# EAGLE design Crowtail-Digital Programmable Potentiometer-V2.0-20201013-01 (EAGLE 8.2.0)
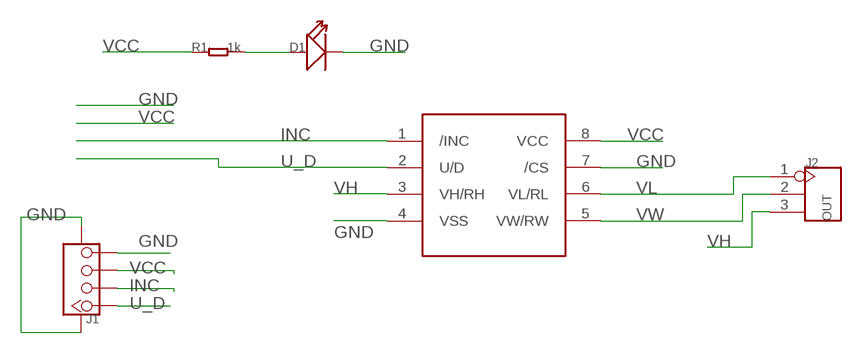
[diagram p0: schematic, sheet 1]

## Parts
D1  LED'0603'  [LED-0603]
J1  TWIG-4P-2.0-SMD-FEMALE-REINFORCE'DD'  [4P-SMD-2.0]
J2  OUT  HEADER-3P-2.54  [3P-2.54]
R1  1k  R-0603  [0603]
U1  X9C103S  [SOP8]

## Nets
GND: D1.- J1.4 J1.SS1 J1.SS2 U1.4(VSS) U1.7(/CS)
INC: J1.2 U1.1(/INC)
N$5: D1.+ R1.2
U_D: J1.1 U1.2(U/D)
VCC: J1.3 R1.1 U1.8(VCC)
VH: J2.3 U1.3(VH/RH)
VL: J2.1 U1.6(VL/RL)
VW: J2.2 U1.5(VW/RW)

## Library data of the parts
D1 = Discrete:LED*
J1 = Connector:TWIG-4P-2.0-SMD-FEMALE-REINFORCE
J2 = Connector:HEADER-3P
R1 = Discrete:R*
U1 = IC:X9C103S

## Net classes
0 default: width 0.203 mm, drill 0.305 mm, clearance 0.152 mm

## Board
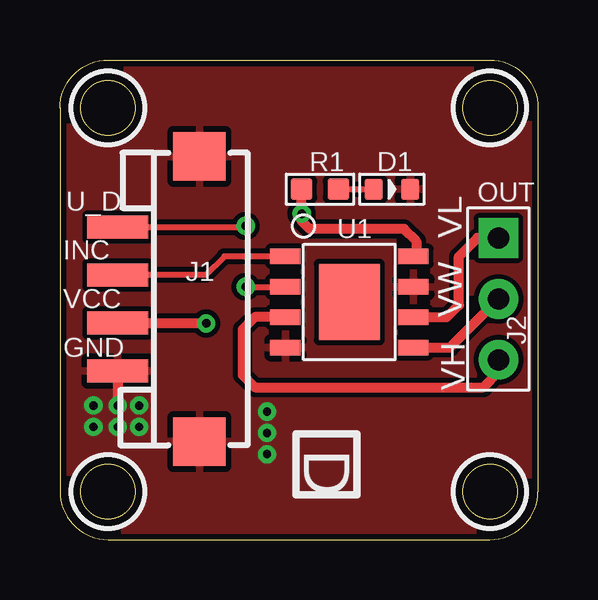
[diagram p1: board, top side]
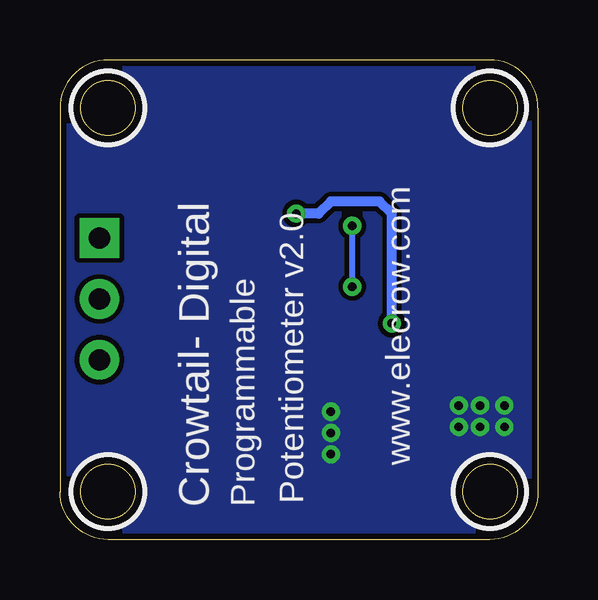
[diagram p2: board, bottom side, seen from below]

Size 19.93 x 20 mm. Coordinates in mm from the lower left corner, seen from the top.
Outline: 0,18 0,2 arc90 2,0 17.93,0 arc90 19.93,2 19.93,18 arc90 17.93,20 2,20 arc90 0,18
Outline: circle at 2,18 radius 1.14
Outline: circle at 2,18 radius 1.14
Outline: circle at 2,2 radius 1.14
Outline: circle at 17.93,18 radius 1.14
Outline: circle at 17.93,18 radius 1.14
Outline: circle at 17.93,2 radius 1.14
Outline: circle at 17.93,2 radius 1.14
Copper layers (1*16): Top 0.035mm / dielectric 1.5mm / Bottom 0.035mm
Design rules "default": minimum track width 10mil, minimum drill 10mil, track to track 8mil, track to pad 8mil, pad to pad 8mil, via to via 8mil, smd to smd 8mil, copper to edge 10mil, drill to drill 8mil, minimum pad ring 10mil, minimum via ring 8mil, stop-mask expansion 4mil, vias tented up to drill 100mil, thermal gap 10mil
tRestrict: area 0.5,16.5 to 3.5,19.5; area 0.5,0.5 to 3.5,3.5; area 16.4,16.5 to 19.5,19.5; area 16.4,0.5 to 19.5,3.5
bRestrict: area 0.5,16.5 to 3.5,19.5; area 0.5,0.5 to 3.5,3.5; area 16.4,16.5 to 19.5,19.5; area 16.4,0.5 to 19.5,3.5

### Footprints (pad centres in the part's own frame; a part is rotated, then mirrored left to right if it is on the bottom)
LED-0603 = smd 0.762 x 0.889: + -0.762,0; - 0.762,0
4P-SMD-2.0 = smd 0.965 x 2.54: 1 -3,0; 2 -1,0; 3 1,0; 4 3,0 | smd 2.032 x 2.184: SS1 -5.946,3.4; SS2 5.946,3.4
3P-2.54 = drill 0.889 pad 1.651 square: 1 0,2.54 | drill 0.889 pad 1.651: 2 0,0; 3 0,-2.54
0603 = smd 0.889 x 0.889: 1 -0.762,0; 2 0.762,0
SOP8 = smd 0.635 x 1.27: 1 -1.905,-2.667; 2 -0.635,-2.667; 3 0.635,-2.667; 4 1.905,-2.667; 5 1.905,2.667; 6 0.635,2.667; 7 -0.635,2.667; 8 -1.905,2.667 | smd 3.175 x 2.54: HEAT 0,0

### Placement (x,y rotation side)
D1  13.84,14.61 0 top
J1  2.41,10.03 270 top
J2  18.29,10.03 0 top
R1  10.84,14.61 0 top
U1  12.06,9.91 270 top

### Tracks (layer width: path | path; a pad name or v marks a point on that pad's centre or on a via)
GND  (via drill 0.35)
  Top 0.406: J1.4 v2.41,5.59
  other vias: 1.4,5.59 3.3,5.59 1.4,4.7 2.41,4.7 3.3,4.7 8.64,5.33 8.64,4.45 8.64,3.56
  pour Top: -0.76,20.83 20.83,20.83 20.83,-0.64 -0.76,-0.64
  pour Bottom: -0.64,20.7 20.7,20.7 20.7,-0.51 -0.64,-0.51
INC
  Top 0.254: J1.2 6.08,11.03 6.86,11.81 U1.1
N$5
  Top 0.254: R1.2 D1.+
U_D  (via drill 0.35)
  Top 0.254: J1.1 7.7,13.03 v7.75,13.08 | v7.75,10.54 U1.2
  Bottom 0.254: v7.75,13.08 v7.75,10.54
VCC  (via drill 0.35)
  Top 0.406: U1.8 14.86,11.94 14.86,12.45 14.35,12.95 10.41,12.95 10.08,13.29 v10.08,13.59 R1.1 | J1.3 6.08,9.03 v6.1,9.02
  Bottom 0.406: v6.1,9.02 6.1,13.59 6.6,14.1 8.64,14.1 9.14,13.59 v10.08,13.59
VH
  Top 0.406: U1.3 8.13,9.27 7.62,8.76 7.62,6.86 8.13,6.35 17.65,6.35 18.29,6.99 J2.3
VL
  Top 0.406: U1.6 16.13,9.27 16.64,9.78 16.64,11.81 17.4,12.57 J2.1
VW
  Top 0.406: U1.5 16.26,8 J2.2

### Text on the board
tPlace: U_D | INC | VCC | GND | D
bPlace: www.elecrow.com | Potentiometer v2.0 | Programmable | Crowtail- Digital
tNames: OUT | VL | VW | VH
